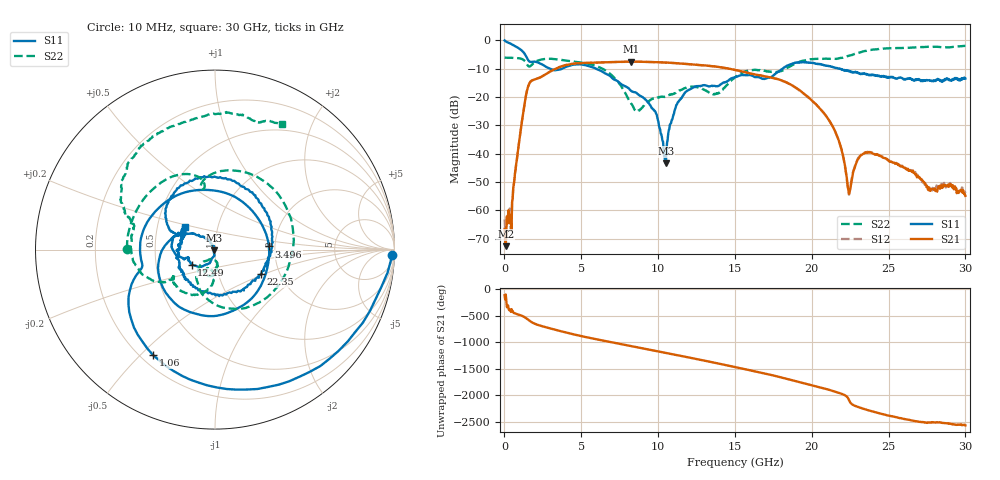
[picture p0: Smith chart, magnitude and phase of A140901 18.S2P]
!  2-Port S-parameters saved by WinCal
! VAR MeasName=S-Parameters (CALIBRATED_DATA) read from VNA (N5244A)
! VAR MeasDate=11/3/2014 9:28:16 AM
! VAR NAME=A140901 18
! VAR FILENAME=A140901 18.S2P
! VAR DATE=11/3/2014 9:28:16 AM
! VAR PHYS_PORTS=1,2
# Hz S RI R 50
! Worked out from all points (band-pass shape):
!   801 points, 10 MHz to 30 GHz, reference 50 ohm
!   highest |S21| = -7.54 dB at 8.257 GHz (marker M1); lowest = -72.6 dB at 84.97 MHz (marker M2)
!   |S21| within 3 dB of the highest: 3.146 GHz to 15.07 GHz (11.92 GHz wide, 131 % of centre)
!   lowest |S11| = -43.4 dB at 10.51 GHz (marker M3), VSWR 1.01, Z = 49.4 - j0.374 ohm
!   |S11| at or under -10 dB: 2.945 GHz to 3.779 GHz (833.8 MHz wide, 24.8 % of centre); 5.93 GHz to 18.12 GHz (12.19 GHz wide, 101 % of centre); 21.76 GHz to end of sweep
!   |S22| runs from -25.1 to -2.0 dB; largest |S21 - S12| = 0.0041
!   S11 on the Smith chart (normalised r, x): 10 MHz: 21, -57; 1.06 GHz: 0.25, -0.54; 3.496 GHz: 1.85, +0.07; 12.49 GHz: 0.76, -0.13; 22.35 GHz: 1.61, -0.48; 30 GHz: 0.69, +0.18
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1e7  0.988 -0.0305  -0.0002 -0.000427  0.000475 0.000507  -0.4906 0.004
8.4975e7  0.9267 -0.2087  -5.62e-05 -0.000227  -0.000319 -0.00017  -0.4895 0.0383
4.223625e8  0.5257 -0.6822  0.000204 -0.000567  0.000251 -0.000358  -0.4517 0.188
1.05965e9  -0.3462 -0.5867  -0.0182 -0.0189  -0.0182 -0.0189  -0.2479 0.4032
1.65945e9  -0.405 -0.0934  -0.0799 0.1613  -0.0798 0.1614  -0.0728 0.3374
2.671612e9  -0.09 0.3321  0.2491 0.0105  0.2492 0.0107  0.2207 0.4118
3.496338e9  0.2999 0.0179  0.1584 -0.2878  0.1588 -0.2875  0.4185 0.1855
5.033325e9  -0.2286 -0.2945  -0.3869 -0.0809  -0.3871 -0.0797  0.3299 -0.2279
6.682775e9  -0.2411 0.0623  -0.03 0.4074  -0.0303 0.4065  -0.0427 -0.2751
8.25725e9  -0.0978 0.0806  0.4182 0.0341  0.4169 0.0345  -0.0445 -0.0609
1.001916e10  -0.0193 0.0311  -0.0376 -0.4075  -0.0376 -0.4066  0.00544 -0.0975
1.05065e10  -0.00562 -0.00378  -0.2202 -0.3385  -0.2195 -0.338  0.00638 -0.1001
1.121876e10  -0.0245 -0.0692  -0.3773 -0.1091  -0.3773 -0.109  0.00778 -0.1213
1.249334e10  -0.1307 -0.0832  -0.199 0.3094  -0.1988 0.3105  -0.0487 -0.141
1.5005e10  -0.2206 -0.0245  0.2623 -0.1446  0.2591 -0.1465  -0.0339 -0.2194
1.721676e10  -0.2026 0.0793  -0.2186 -0.0476  -0.2176 -0.047  -0.236 -0.1536
2.002832e10  0.0871 0.3903  0.0833 -0.0185  0.0834 -0.0174  -0.4603 -0.0377
2.16028e10  0.3185 0.0468  -0.0164 -0.0147  -0.0161 -0.0148  -0.4492 0.1307
2.235255e10  0.2577 -0.1353  -0.000882 0.00236  -0.00068 0.00237  -0.4911 0.1891
2.328974e10  0.0522 -0.2475  0.000435 -0.00966  0.000346 -0.0099  -0.5235 0.3476
2.501416e10  -0.1833 -0.116  -0.00535 0.00507  -0.00557 0.00533  -0.334 0.6389
3e10  -0.1673 0.127  0.0012 -0.00134  0.00124 -0.00158  0.3737 0.7009
